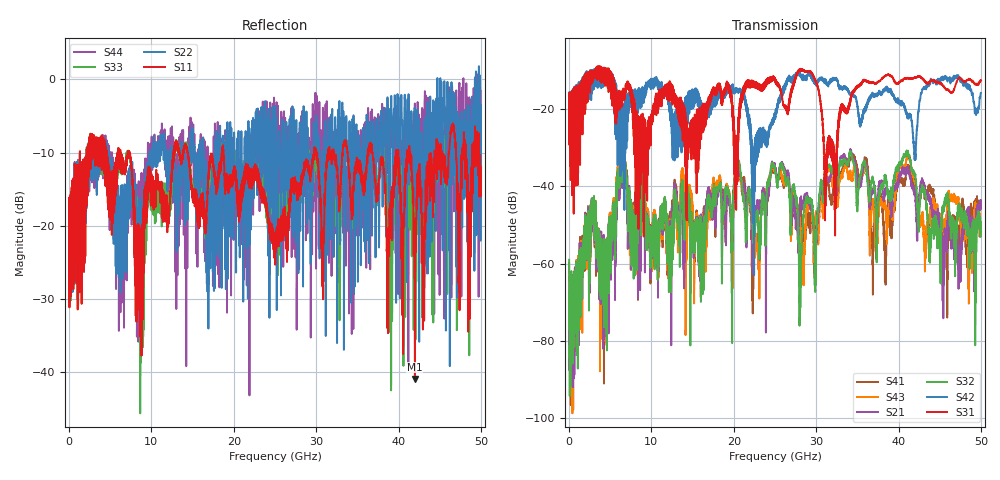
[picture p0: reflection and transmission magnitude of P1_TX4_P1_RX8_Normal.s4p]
!Keysight Technologies,N5225B,MY57041031,A.13.20.10
!Date: Friday, May 31, 2019 11:25:55
!Correction: S11(Full 4 Port(1,2,3,4))
!S12(Full 4 Port(1,2,3,4))
!S13(Full 4 Port(1,2,3,4))
!S14(Full 4 Port(1,2,3,4))
!S21(Full 4 Port(1,2,3,4))
!S22(Full 4 Port(1,2,3,4))
!S23(Full 4 Port(1,2,3,4))
!S24(Full 4 Port(1,2,3,4))
!S31(Full 4 Port(1,2,3,4))
!S32(Full 4 Port(1,2,3,4))
!S33(Full 4 Port(1,2,3,4))
!S34(Full 4 Port(1,2,3,4))
!S41(Full 4 Port(1,2,3,4))
!S42(Full 4 Port(1,2,3,4))
!S43(Full 4 Port(1,2,3,4))
!S44(Full 4 Port(1,2,3,4))
!S4P File: Measurements: <S11,S12,S13,S14>,
!<S21,S22,S23,S24>,
!<S31,S32,S33,S34>,
!<S41,S42,S43,S44>:
# Hz S  dB  R 50.0
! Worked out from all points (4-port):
!   5000 points, 10 MHz to 50 GHz, reference 50 ohm
!   strongest paths, dB at 10 MHz, 12.51 GHz, 25.01 GHz, 37.51 GHz, 50 GHz:
!     S31: -19.6, -17.6, -12.9, -13.1, -12.6
!     S42: -19.4, -24.4, -22.6, -16.2, -15.9
!     S32: -59.0, -55.5, -35.9, -46.5, -50.8
!     S21: -59.9, -50.1, -35.0, -42.7, -43.6
!     S43: -63.6, -48.3, -36.2, -48.3, -50.4
!     S41: -64.9, -45.7, -36.1, -47.3, -44.1
!   lowest |S11| = -40.9 dB at 41.99 GHz (marker M1), VSWR 1.02, Z = 50.9 - j0.00886 ohm
!   |S11| at or under -10 dB: 7.336 GHz to 12.7 GHz (5.362 GHz wide, 53.5 % of centre); 14.42 GHz to 18.57 GHz (4.155 GHz wide, 25.2 % of centre); 18.74 GHz to 29.76 GHz (11.02 GHz wide, 45.4 % of centre)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
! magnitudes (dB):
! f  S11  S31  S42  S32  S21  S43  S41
! 10 MHz  -19.5  -19.6  -19.4  -59.0  -59.9  -63.6  -64.9
! 6.44 GHz  -12.1  -15.7  -30.3  -31.3  -32.8  -30.4  -31.5
! 25.81 GHz  -21.2  -16.2  -16.6  -34.0  -33.7  -36.9  -37.3
! 28.1 GHz  -14.4  -9.9  -11.2  -61.2  -44.2  -52.6  -45.7
! 32.24 GHz  -10.4  -35.6  -12.0  -37.9  -37.0  -38.8  -38.2
! 41.99 GHz  -40.9  -11.9  -32.6  -37.0  -41.4  -38.3  -41.4
! 50 GHz  -12.0  -12.6  -15.9  -50.8  -43.6  -50.4  -44.1
